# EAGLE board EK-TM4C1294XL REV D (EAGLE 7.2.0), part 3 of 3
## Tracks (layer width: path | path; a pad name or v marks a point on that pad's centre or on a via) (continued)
PQ3  (via drill 0.3) (continued)
  Bottom 0.152: v45.41,12.57 45.41,12.04 45.49,11.96 45.49,10.97 44.42,9.91 44.42,8.99 44.5,8.91 X7.14 | v49.68,34.29 49.68,34.82 49.53,34.98 49.53,37.8 49.76,38.02 49.76,39.09 49.84,39.17 v49.84,39.32 | v44.81,33.83 43.81,32.84 43.81,32 44.81,31.01 44.81,28.5 44.12,27.81 44.12,25.91 44.2,25.83 44.2,25.6 44.73,25.07 44.73,22.94 45.34,22.25 45.34,16.31 44.81,15.77 44.81,15.32 45.41,14.71 v45.41,12.57 | 45.41,12.5 v45.41,12.57 | X11.57 52.07,5.84 v50.6,7.32
PQ4  (via drill 0.3)
  Top 0.152: U4.5 81.31,41.45 81.46,41.3 82.6,41.3 82.83,41.53 82.83,41.6 v82.91,41.68 | v79.48,17.98 78.94,17.98 78.18,17.22 76.2,17.22 75.89,17.53 73.53,17.53 73.08,17.98 v69.49,17.98 68.73,17.98 68.66,18.06 52.27,18.06 51.66,18.67 49,18.67 48.08,19.58 47.55,19.58 46.94,18.97 43.81,18.97 43.05,18.21 38.25,18.21 37.03,16.99 27.74,16.99 26.52,18.21 23.62,21.03 16.38,21.03 11.73,16.38 11.73,13.87 11.73,12.34 10.9,11.51 10.59,11.51 9.37,11.51 8.46,11.51 8,10.9 v6.25,10.9 | v69.11,21.79 58.37,21.79 57.68,22.48 51.82,22.48 51.07,23.23 U1.P$102
  Bottom 0.152: v82.91,41.68 82.83,41.68 81.08,39.93 81.08,33.6 | 81.08,33.6 81.15,33.53 | 81.08,33.6 81.08,19.58 v79.48,17.98 | X11.93 6.33,4.27 6.33,4.8 6.2,4.93 6.2,10.16 6.25,10.21 v6.25,10.9 | v69.11,21.79 69.49,21.41 v69.49,17.98
RBIAS
  Top 0.152: R25.1 37.72,35.74 38.71,34.75 39.57,34.75 U1.P$59
TARGET_ID  (via drill 0.3)
  Top 0.152: U2.2 6.55,24.13 v6.53,24.11 | R18.2 16.99,22.78 16.76,22.55 13.79,22.55 13.03,21.79 13.03,20.65 TP7.TP 8.46,22.02 v6.93,22.02 5.78,23.18 U7.P4
  Bottom 0.152: v6.53,24.11 6.63,24.08 6.63,23.01 6.93,22.71 v6.93,22.02
TARGET_RXD
  Top 0.152: X1.12 R7.1 82.37,26.52 82.34,26.48 82.34,26.25 81.84,25.76 76.56,25.76 JP4.1
TARGET_TCK/SWCLK
  Top 0.152: X1.10 R8.1 82.37,23.62 82.14,23.39 80.09,23.39 79.78,23.7 78.72,23.7 75.82,20.8 68.12,20.8 67.82,21.11 57.91,21.11 57.15,21.87 54.86,21.87 54.79,21.79 54.79,21.2 R1.2 54.69,21.11 51.44,21.11 51.13,21.41 51.13,22.06 U1.P$100
TARGET_TDI
  Top 0.152: X1.6 R11.1 82.37,18.97 82.37,18.52 82.34,18.48 82.14,18.29 80.7,18.29 78.41,20.57 77.04,20.57 75.74,19.28 72.85,19.28 72.62,19.51 68.58,19.51 68.05,18.97 52.96,18.97 52.35,19.58 50.98,19.58 50.52,20.04 50.52,21.54 U1.P$98
TARGET_TDO/SWO  (via drill 0.3)
  Top 0.152: X1.4 R15.1 82.45,16.38 82.45,16.08 82.14,15.77 v74.83,15.77 | v74.83,18.67 72.92,18.67 72.47,19.13 68.81,19.13 68.35,18.67 52.73,18.67 52.12,19.28 49.45,19.28 49.07,19.66 49.07,21.26 U1.P$97
  Bottom 0.152: v74.83,18.67 v74.83,15.77
TARGET_TMS/SWDIO
  Top 0.152: X1.8 R10.1 82.37,21.57 82.37,21.03 82.14,20.8 79.25,20.8 78.64,21.41 76.89,21.41 75.97,20.5 67.74,20.5 67.44,20.8 57.91,20.8 56.69,19.58 54.86,19.58 54.77,19.68 R2.2 54.67,20.34 51.21,20.34 50.83,20.73 50.83,21.79 U1.P$99
TARGET_TXD  (via drill 0.3)
  Top 0.152: R6.1 X1.14 | JP5.1 85.01,31.75 v85.11,31.85
  Bottom 0.152: v85.11,31.85 85.11,29.23 X1.14
TARGET_VBUS  (via drill 0.3)
  Top 0.152: 9.04,24.64 v9.14,24.54 | X11.60 48.49,1.27 47.32,2.44 v43.28,2.44 | v13.72,21.03 14.17,21.49 14.17,21.72 14.55,22.1 21.34,22.1 21.49,22.25 26.21,22.25 30.56,17.91 36.27,17.91 37.49,19.13 42.37,19.13 43.59,20.34 v44.42,20.34 44.88,20.8 46.46,20.8 U1.P$96
  Top 0.254: 9.04,24.64 U2.6
  Top 0.356: 81.74,42.09 U4.6
  Top 0.381: JP1.3 73.69,43.2 75.36,43.2 76.2,44.04 81.61,44.04 v81.84,43.89 | v81.84,41.99 81.74,42.09 | v36.96,34.67 32.69,34.67 30.94,36.42 27.81,36.42 25.22,33.83 23.62,33.83 21.95,32.16 13.34,32.16 11.43,30.25 TP4.TP 7.09,26.67 5.52,25.11 5.5,25.12 U7.P1 | v70.87,48.92 68.2,48.92 66.52,47.24 55.78,47.24 55.02,46.56 47.09,46.56 46.79,46.86 39.55,46.86 39.09,46.41 v38.56,46.41
  Bottom 0.152: v9.14,24.54 9.14,25.65 TP4.TP 11.46,27.96 13.03,27.96 13.95,27.05 13.95,24.69 13.72,24.46 v13.72,21.03 | v43.28,2.44 43.28,6.33 42.14,7.47 42.14,7.54 43.05,8.46 43.05,11.58 43.28,11.81 43.28,15.24 44.42,16.38 v44.42,20.34
  Bottom 0.381: v81.84,43.89 81.53,43.59 81.53,42.29 v81.84,41.99 | v36.96,34.67 37.26,34.98 37.26,38.94 39.78,41.45 39.78,42.22 38.56,43.43 v38.56,46.41 | v70.87,48.92 70.87,43.43 JP1.3
TARGET_VDDC
  Top 0.152: TP12.TP 62.26,24.16 | 54.75,26.93 U1.P$115
  Top 0.229: 54.75,26.93 55.4,26.29
  Top 0.254: C4.1 41.53,23.55 41.91,23.16 43.74,23.16 43.74,23.18 U1.P$87 47.99,27.43 49.3,27.43 49.99,26.75 51.05,26.75 52.43,28.12 53.11,28.12 53.49,27.74 53.94,27.74 U1.P$115 | 55.4,26.29 56.83,26.29 C15.1 | C14.1 57.99,25.15 57.8,25.34 57.8,25.48 C15.1 | TP12.TP 62.23,26.01 61.65,26.59 58.52,26.59 57.84,25.91 C15.1
USBD_N
  Top 0.203: 45.96,22.01 U1.P$93
  Top 0.229: 45.95,22.01 45.96,22.01
  Top 0.275: 45.95,22.01 42.58,22.01 40.83,20.25 35.06,20.25 34.3,21.02 30.72,21.02 27.67,24.06 13.34,24.06 13.34,24.13 TP5.TP 10.16,25.4 7.77,25.4 7.42,25.04 U2.1 6.99,24.64 6.83,24.79 6.22,24.79 5.89,24.46 5.88,24.48 U7.P2
USBD_P
  Top 0.203: 45.95,21.58 46.1,21.58 U1.P$94
  Top 0.275: 45.95,21.58 42.76,21.58 41.01,19.83 34.89,19.83 34.12,20.59 30.54,20.59 27.5,23.64 13.34,23.64 13.34,23.5 TP6.TP 10.16,22.86 7.77,22.86 7.39,23.24 U2.3 6.99,23.62 6.86,23.5 6.86,23.47 6.78,23.39 6.33,23.39 6.25,23.47 6.2,23.5 5.87,23.82 U7.P3
VBAT  (via drill 0.3)
  Top 0.152: R38.1 33.15,28.79 33.22,28.8 | 33.22,28.8 32.69,28.8 32.38,29.11 32,29.11 31.93,29.18 31.85,29.17 R42.1 | 33.22,28.8 33.3,28.8 33.3,29.34 v33.76,29.79 | R39.1 31.93,22.48 31.93,23.24 31.76,23.41 31.76,23.5 TP11.TP
  Bottom 0.152: v33.76,29.79 33.76,26.14 TP11.TP
VBUS
  Top 0.152: R36.2 79.9,39.9 79.86,39.85 R35.1 | R35.1 78.88,39.87 78.26,39.24 77.04,39.24 76.73,39.55 75.11,39.55 JP1.6 | R35.1 79.65,39.84 R35.1
  Top 0.356: U4.2 77.04,42.75 76.2,41.91
  Top 0.381: 76.2,41.91 JP1.4 | 74.95,39.4 JP1.6
  Bottom 0.381: JP1.2 JP1.4 JP1.6
VCP_RXD  (via drill 0.3)
  Top 0.152: R6.2 82.31,30.25 86.56,30.25 87.61,29.21 X1.13 87.66,29.18 90.22,29.18 91.59,27.81 96.09,27.81 97.46,29.18 v99.67,29.18 | U20.P$17 105.45,24.53 105.08,24.16 103.78,24.16 100.66,27.28 v99.67,27.28
  Bottom 0.152: v99.67,29.18 v99.67,27.28
VCP_TXD
  Top 0.152: R7.2 82.26,27.66 86.79,27.66 87.63,26.82 X1.11 87.71,26.75 99.21,26.75 99.36,26.59 100.81,26.59 103.56,23.85 105.31,23.85 105.95,24.5 U20.P$18
VERSION_0  (via drill 0.3)
  Top 0.152: v104.09,43.97 104.09,44.65 104.1,44.66 104.01,44.74 R12.1 | v105.39,39.47 105.99,38.86 105.99,38.79 106.95,37.83 U20.P$61
  Bottom 0.152: v105.39,39.47 104.09,40.77 v104.09,43.97
VERSION_1  (via drill 0.3)
  Top 0.152: U20.P$47 114.85,34.37 113.46,34.37 112.32,33.22 v108.89,33.22 | v105.16,43.97 105.18,43.84 R13.1
  Bottom 0.152: v105.16,43.97 105.16,43.05 105.99,42.22 105.99,36.12 v108.89,33.22
VERSION_2  (via drill 0.3)
  Top 0.152: U20.P$48 114.88,34.9 113.16,34.9 111.94,33.68 109.5,33.68 v108.97,34.21 | v106.38,43.97 106.35,43.84 R14.1
  Bottom 0.152: v108.97,34.21 106.38,36.8 v106.38,43.97
VREF+  (via drill 0.3)
  Top 0.152: v84.05,32.69 81.53,32.69 81.38,32.84 72.01,32.84 70.1,34.75 64.29,34.75 63.83,34.29 TP13.TP 62.19,34.33 62.26,34.29 61.78,34.76 61.55,34.76 60.88,35.43 60.88,35.89 60.81,35.97 R41.1 60.1,36.02 59.66,35.59 56.71,35.59 U1.P$9
  Bottom 0.152: X11.34 84.05,2.77 v84.05,32.69
VREG_EN  (via drill 0.3)
  Top 0.152: v94.64,34.9 94.03,34.9 93.73,34.59 93.73,33.83 93.8,33.76 R17.2 92.96,33.6 92.28,34.29 TP3.TP
  Top 0.305: U5.4 96.99,39.84 v97.46,40.31
  Bottom 0.152: v97.46,40.31 97.46,39.24 96.47,38.25 94.94,38.25 94.64,37.95 v94.64,34.9

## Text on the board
Bottom: EK-TM4C1294XL / REV D
tPlace: DEBUG | TXD | RXD | Target USB | TCK | TMS | TDI | BoosterPack 2 | TDO | BoosterPack 1 | !RESET | TM | Tiva C Series / Connected LaunchPad | 85 | 71 | 57 | 43 | 29 | 15 | 1
bPlace: TXD | RXD | TCK | TMS | TDI | TDO | !RESET
tNames: POWER | http://www.ti.com/launchpad | POWER SELECT | U22 | BoosterPack | +3v3 | OTG | ICDI | U14 | CAN | UART | MCU 3V3 | Y2 | CAN | Y1 | UART | EK-TM4C1294XL Rev D
bNames: +3v3 / PD2 / PP0 / PP1 / See JP4 / See JP5 / PQ0 / PP4 / PN5 / PN4 | +5V / GND / PB4 / PB5 / PK0 / PK1 / PK2 / PK3 / PA4 / PA5 | TP1 | TP8 | +3V3 / PE4 / PC4 / PC5 / PC6 / PE5 / PD3 / PC7 / PB2 / PB3 | TP10 | TP13 | TP3 | +5V / GND / PE0 / PE1 / PE2 / PE3 / PD7 / PA6 / PM4 / PM5 | TP9 | BP2_A2.6 / PA1 | PD5 / ICDI_TX | TP4 | TP5 | PG1 / PK4 / PK5 / PM0 / PM1 / PM2 / PH0 / PH1 / PK6 / PK7 | TP12 | BP2_A2.5 / PA0 | PD4 / ICDI RX | TP2 | TP6 | TP11 | PF1 / PF2 / PF3 / PG0 / PL4 / PL5 / PL0 / PL1 / PL2 / PL3 | TP7 | GND / PM7 / PP5 / PA7 / !RESET / PQ2/PA3 / PQ3/PA2 / PP3 / PQ1 / PM6 | GND / PM3 / PH2 / PH3 / !RST / PD1 / PD0 / PN2 / PN3 / PP2 | 5V / 3V3 | !WAK / GND | PQ4 / !RST | PN3 / PM4 | PN2 / PM5 | PN1 / PM6 | PN0 / PM7 | PN5 / PJ1 | PN4 / PJ0 | PL5 / PP5 | PK4 / PP4 | PK5 / PA1 | PP3 / PA0 | PP2 / PF3 | PB3 / PF2 | PB2 / PF1 | PL4 / PF0 | PK6 / PF4 | GND / GND | PK7 / PB1 | PQ3 / PB0 | PQ2 / PP1 | PQ1 / PP0 | PQ0 / PD2 | PL3 / PD0 | PL2 / PD1 | PL1 / PD3 | PL0 / PD6 | PM0 / PD7 | PM1 / PD4 | PM2 / PD5 | GND / GND | PM3 / REF | PG0 / PK3 | PG1 / PK2 | PA7 / PK1 | PA6 / PK0 | PC4 / PE5 | PC5 / PE4 | PC6 / PE3 | PC7 / PE2 | PH3 / PE1 | PH2 / PE0 | PH1 / PA5 | PH0 / PA4 | PB5 / PA3 | PB4 / PA2 | GND / GND | 3V3 / 5V
Document: Layer Stackup / Top silkscreen / Top Solder Mask / Component Side / Layer 2 / Layer 3 / Solder Side / Bottom Solder Mask / Bottom Silkscreen | File Names / EK-TM4C129EXL.sst / EK-TM4C129EXL.smt / EK-TM4C129EXL.l1 / EK-TM4C129EXL.l2 / EK-TM4C129EXL.l3 / EK-TM4C129EXL.l4 / EK-TM4C129EXL.smb / EK-TM4C129EXL.ssb | NOTES: UNLESS OTHERWISE SPECIFIED / 1) Manufacture in accordance with IPC-6012, Type 3, Class 2. / 2) End Product Features shall not vary more than 20% from artwork originals / 3) Material shall be ROHS compliant, copper clad FR-406, NEMA Grade (Tg 170degC) / Per IPC-4101, Color Natural, or equivalent / 4) Construction shall be symetrical multilayer per layer stackup detail / 5) Copper weight on inner layers shall be 1 oz per square foot / 6) Equivalent copper weight on outler layers shall be 1.0 oz per square foot before plating / 7) All plated through holes shall have a minimum of 0.0007 inches of copper / 8) Drill hole tolerance after plating shall be +/- 0.003 inches / 9) Minimum annular ring shall be 0.001 inches / 10) Minmum annular rint at emergent conductors shall be 0.003 inches / 11) PCB Thickness shall be 0.062 inches +/- 0.007 inches / 12) Warp / Twist shall not exceed 0.010 inches per inch / 13) Finish shall be LPI, Gloss RED SMOBC, Both sides balance of exposed copper shall be HASL / 14) Silkscreen with nonconductive white epoxy ink / 15) Board stack-up should be targetted such that a differential impedance of 90 ohms +/- 10% can / be achieved on the top layer with 10.8 mil traces and 6 mil spacing. Additionally 100 ohm +/- 10% / with 8.7 mil traces and 6 mil spacing. Boards do not need to be impedance controlled.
